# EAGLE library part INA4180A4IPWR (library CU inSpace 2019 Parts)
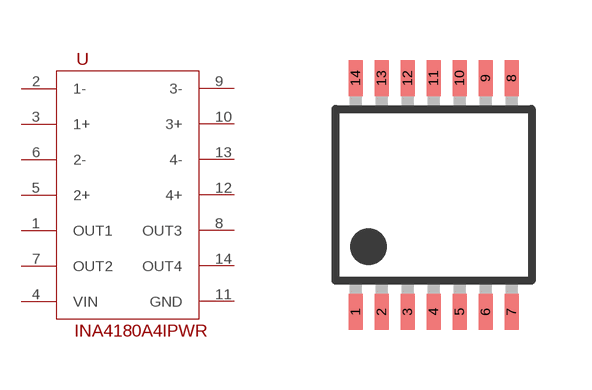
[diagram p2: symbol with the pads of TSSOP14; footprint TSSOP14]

Designator prefix U

## INA4180A4IPWR  [TSSOP14]
1  OUT1
2  1-
3  1+
4  VIN
5  2+
6  2-
7  OUT2
8  OUT3
9  3-
10  3+
11  GND
12  4+
13  4-
14  OUT4

## Footprint TSSOP14 (pad centres in mm)
plastic thin shrink small outline package; 14 leads; body width 4.4 mm SOT402-1 Source: http://www.nxp.com/documents/data_sheet/74ABT125.pdf
smd 0.35 x 0.9: 1 -1.95,-2.925; 2 -1.3,-2.925; 3 -0.65,-2.925; 4 0,-2.925; 5 0.65,-2.925; 6 1.3,-2.925; 7 1.95,-2.925; 8 1.95,2.925; 9 1.3,2.925; 10 0.65,2.925; 11 0,2.925; 12 -0.65,2.925; 13 -1.3,2.925; 14 -1.95,2.925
